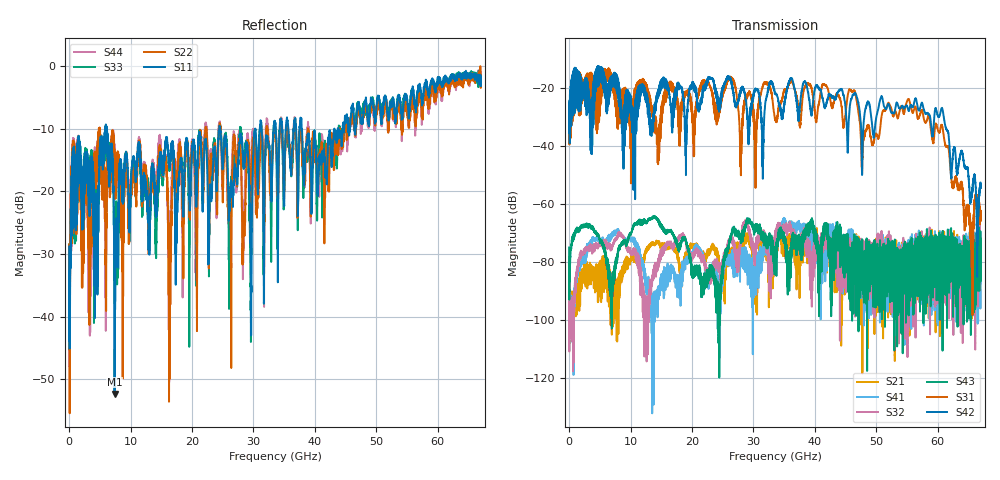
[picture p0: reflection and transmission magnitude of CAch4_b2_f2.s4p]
!Agilent Technologies,N5247A,US51170199,A.09.90.13
!Agilent N5247A: A.09.90.13
!Date: Thursday, October 18, 2018 09:40:35
!Correction: S11(Full 4 Port(1,2,3,4))
!S12(Full 4 Port(1,2,3,4))
!S13(Full 4 Port(1,2,3,4))
!S14(Full 4 Port(1,2,3,4))
!S21(Full 4 Port(1,2,3,4))
!S22(Full 4 Port(1,2,3,4))
!S23(Full 4 Port(1,2,3,4))
!S24(Full 4 Port(1,2,3,4))
!S31(Full 4 Port(1,2,3,4))
!S32(Full 4 Port(1,2,3,4))
!S33(Full 4 Port(1,2,3,4))
!S34(Full 4 Port(1,2,3,4))
!S41(Full 4 Port(1,2,3,4))
!S42(Full 4 Port(1,2,3,4))
!S43(Full 4 Port(1,2,3,4))
!S44(Full 4 Port(1,2,3,4))
!S4P File: Measurements: <S11,S12,S13,S14>,
!<S21,S22,S23,S24>,
!<S31,S32,S33,S34>,
!<S41,S42,S43,S44>:
# Hz S  dB  R 50
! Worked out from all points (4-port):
!   6701 points, 10 MHz to 67 GHz, reference 50 ohm
!   strongest paths, dB at 10 MHz, 16.76 GHz, 33.51 GHz, 50.25 GHz, 67 GHz:
!     S42: -30.4, -28.1, -21.7, -27.7, -53.9
!     S31: -30.6, -21.4, -30.8, -37.3, -63.8
!     S43: -75.0, -70.2, -79.4, -85.3, -75.1
!     S32: -88.9, -74.7, -71.2, -77.8, -80.1
!     S41: -78.0, -83.2, -78.7, -81.1, -76.4
!     S21: -80.7, -74.2, -74.4, -79.3, -74.0
!   lowest |S11| = -52.3 dB at 7.399 GHz (marker M1), VSWR 1.00, Z = 50.1 + j0.233 ohm
!   |S11| at or under -10 dB: start of sweep to 5.859 GHz; 6.124 GHz to 24.42 GHz (18.3 GHz wide, 120 % of centre); 24.6 GHz to 30.25 GHz (5.648 GHz wide, 20.6 % of centre)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
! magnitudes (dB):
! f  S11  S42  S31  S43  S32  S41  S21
! 10 MHz  -28.8  -30.4  -30.6  -75.0  -88.9  -78.0  -80.7
! 7.399 GHz  -52.3  -15.3  -22.5  -82.8  -72.2  -69.1  -84.8
! 16.4 GHz  -14.6  -23.2  -17.9  -69.6  -73.6  -86.6  -75.3
! 45.84 GHz  -8.1  -24.3  -20.8  -91.4  -75.2  -70.7  -78.9
! 47.77 GHz  -9.0  -37.8  -41.3  -80.9  -74.7  -80.2  -98.3
! 55.18 GHz  -6.8  -27.6  -23.9  -73.4  -81.9  -89.8  -88.0
! 67 GHz  -3.2  -53.9  -63.8  -75.1  -80.1  -76.4  -74.0
